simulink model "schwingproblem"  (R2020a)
settings: Solver=ode45  StartTime=0.0  StopTime=100  RelTol=1e-3  EnableMultiTasking=on

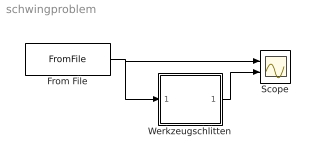
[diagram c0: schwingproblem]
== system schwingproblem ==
  From File : FromFile  FileName=schwingung.mat  SampleTime=0
  Scope : Scope  NumInputPorts=2
  Werkzeugschlitten : Subsystem  mask(Schwingkreis){D=0.001, om0=50, b0=40}
      mask prompts: D "Daempfungsgrad"; om0 "Eigenfrequenz"; b0 "Staerke"
      mask help: Harmonischer Schwinger mit Eigenfrequenz omega0 und Daempfungsgrad D. Die Erregerfunktion werde mit einer Verstaerkung eingekoppelt.
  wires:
  From File/1 -> Werkzeugschlitten/1(u), Scope/1
  Werkzeugschlitten/1(x) -> Scope/2

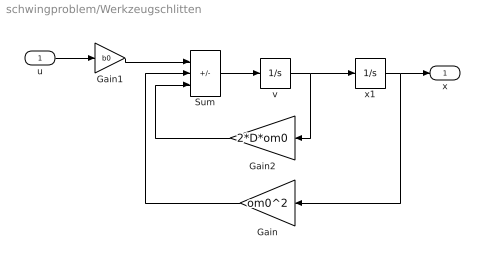
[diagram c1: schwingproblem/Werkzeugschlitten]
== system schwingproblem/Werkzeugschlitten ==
  u : Inport
  Gain : Gain  Gain=om0^2  SaturateOnIntegerOverflow=on
  Gain1 : Gain  Gain=b0  SaturateOnIntegerOverflow=on
  Gain2 : Gain  Gain=2*D*om0  SaturateOnIntegerOverflow=on
  Sum : Sum  Inputs=+--  SaturateOnIntegerOverflow=on
  v : Integrator
  x1 : Integrator
  x : Outport
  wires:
  Sum/1 -> v/1
  v/1 -> x1/1, Gain2/1
  Gain1/1 -> Sum/1
  x1/1 -> x/1, Gain/1
  u/1 -> Gain1/1
  Gain2/1 -> Sum/3
  Gain/1 -> Sum/2
